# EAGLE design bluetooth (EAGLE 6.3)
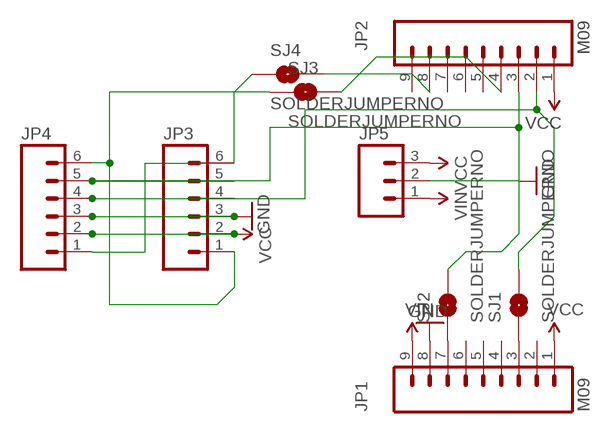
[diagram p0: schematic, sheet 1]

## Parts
JP1  M09  [1X09]
JP2  M09  [1X09]
JP3  M06LOCK  [1X06_LOCK]
JP4  M06LOCK  [1X06_LOCK]
JP5  M03PTH  [1X03]
SJ1  SOLDERJUMPERNO  [SJ_2S-NO]
SJ2  SOLDERJUMPERNO  [SJ_2S-NO]
SJ3  SOLDERJUMPERNO  [SJ_2S-NO]
SJ4  SOLDERJUMPERNO  [SJ_2S-NO]

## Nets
GND [POWER]: JP1.8 JP3.3 JP4.3 JP5.2
N$1: JP2.2 JP3.4 JP4.4 SJ1.2
N$2: JP2.3 JP3.5 JP4.5 SJ2.2
N$3: JP1.3 SJ1.1
N$4: JP1.7 SJ2.1
N$5: JP3.6 JP4.1 SJ4.1
N$6: JP3.1 JP4.6 SJ3.1
N$7: JP2.8 SJ4.2
N$8: JP2.4 SJ3.2
VCC: JP1.1 JP2.1 JP3.2 JP4.2 JP5.3
VIN: JP1.9 JP5.1
Unconnected: JP1.2 JP1.4 JP1.5 JP1.6 JP2.5 JP2.6 JP2.7 JP2.9

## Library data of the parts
JP1 JP2 = SparkFun:M09: Header 9 Standard 9-pin 0.1" header. Use with straight break away headers (SKU : PRT-00116), right angle break away headers (PRT-00553), swiss pins (PRT-00743), machine pins (PRT-00117), and female headers (PRT-00115).
JP3 JP4 = SparkFun-Connectors:M06: Header 6 Standard 6-pin 0.1" header. Use with straight break away headers (SKU : PRT-00116), right angle break away headers (PRT-00553), swiss pins (PRT-00743), machine pins (PRT-00117), and female headers (PRT-00115). Molex polarized connector foot print use with SKU : PRT-08094 with associated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
JP5 = SparkFun:M03: Header 3 Standard 3-pin 0.1" header. Use with straight break away headers (SKU : PRT-00116), right angle break away headers (PRT-00553), swiss pins (PRT-00743), machine pins (PRT-00117), and female headers (PRT-00115). Molex polarized connector foot print use with SKU : PRT-08232 with associated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
SJ1-SJ4 = SparkFun-Passives:SOLDERJUMPER: Solder Jumper

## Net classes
1 POWER: width 0.203 mm

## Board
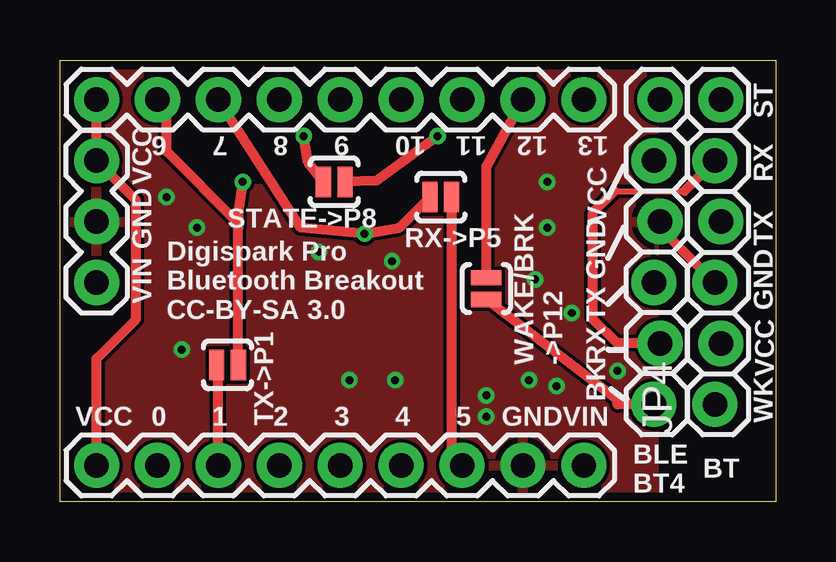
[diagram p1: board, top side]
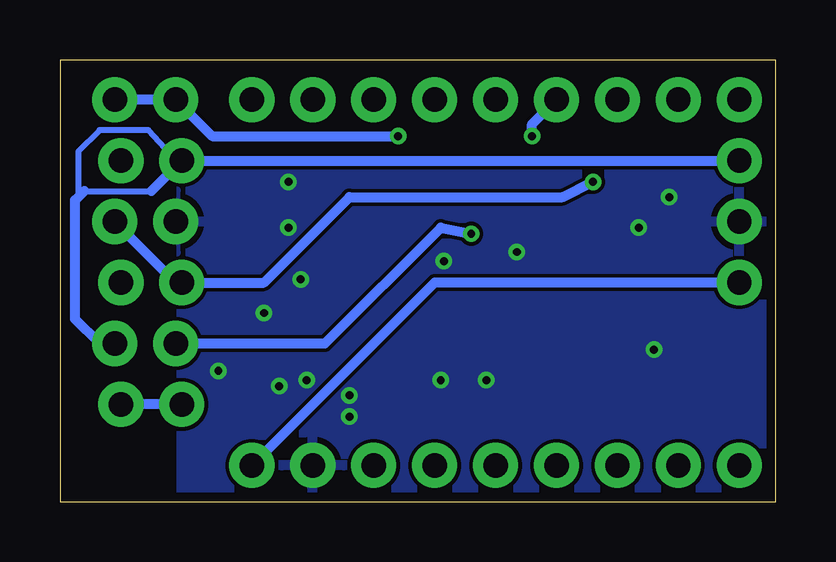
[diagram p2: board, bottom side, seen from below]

Size 29.84 x 18.41 mm. Coordinates in mm from the lower left corner, seen from the top.
Outline: 0,0 0,18.41 29.84,18.41 29.84,0 0,0
Copper layers (1*16): Top 0.0356mm / dielectric 1.5011mm / Bottom 0.0356mm
Design rules "eriks": minimum track width 6mil, minimum drill 13mil, track to track 6mil, track to pad 6mil, pad to pad 6mil, via to via 6mil, smd to smd 6mil, copper to edge 15mil, drill to drill 6mil, minimum pad ring 7mil, minimum via ring 7mil, stop-mask expansion 4mil, vias tented up to drill 20mil, thermal gap 10mil

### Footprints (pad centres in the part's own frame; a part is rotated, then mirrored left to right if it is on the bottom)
1X09 = drill 1.016 pad 1.88: 1 0,0; 2 2.54,0; 3 5.08,0; 4 7.62,0; 5 10.16,0; 6 12.7,0; 7 15.24,0; 8 17.78,0; 9 20.32,0
1X06_LOCK = drill 1.016 pad 1.88: 1 0,0; 2 2.54,-0.254; 3 5.08,0; 4 7.62,-0.254; 5 10.16,0; 6 12.7,-0.254
1X03 = drill 1.016 pad 1.88: 1 0,0; 2 2.54,0; 3 5.08,0
SJ_2S-NO = smd 0.635 x 1.27: 1 -0.45,0; 2 0.45,0

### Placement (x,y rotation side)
JP1  1.52,1.52 0 top
JP2  1.52,16.76 0 top
JP3  25.02,16.76 270 top
JP4  27.3,4.06 90 top
JP5  1.52,9.14 90 top
SJ1  6.99,5.71 0 top
SJ2  15.88,12.7 180 top
SJ3  11.43,13.34 180 top
SJ4  17.78,8.89 90 top

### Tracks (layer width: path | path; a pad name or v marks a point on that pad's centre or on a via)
GND  (via drill 0.33)
  Top 0.406: JP3.3 25.02,11.43 JP4.3
  other vias: 20.32,11.43 13.97,5.08 12.06,5.08 10.79,10.41 4.45,12.7 20.32,13.34 5.71,11.43 5.08,6.35 21.34,7.87 19.81,9.27 23.24,5.46 20.7,4.83 19.56,5.08 17.78,4.45 17.78,3.56 13.84,10.03
  pour Top: -2.54,24.13 -2.54,-1.91 24.77,-1.91 24.77,24.13
  pour Bottom: -2.54,23.5 -2.54,-2.54 24.77,-2.54 24.77,23.5
N$1  (via drill 0.33)
  Top 0.406: SJ1.2 7.43,11.43 | 7.43,11.43 7.43,11.62 4.45,14.61 4.45,16.38 JP2.2 | v7.62,13.34 7.43,12.06 7.43,11.43
  Bottom 0.406: JP4.4 25.02,9.14 JP3.4 21.34,9.14 17.78,12.7 8.89,12.7 v7.62,13.34
N$2  (via drill 0.33)
  Top 0.254: 23.11,12.95 26.04,12.95
  Top 0.406: JP2.3 10.03,11.43 v12.7,11.18 14.15,11.43 SJ2.2 | JP3.5 23.24,6.6 22.23,7.62 22.23,12.06 22.86,12.7 23.11,12.95 | 26.04,12.95 JP4.5
  Bottom 0.406: JP3.5 18.8,6.6 13.97,11.43 v12.7,11.18
N$3
  Top 0.406: JP1.3 6.6,5.65 SJ1.1
N$4
  Top 0.406: SJ2.1 16.32,1.96 JP1.7
N$5
  Top 0.406: JP3.6 23.24,4.06 23.24,4.25 SJ4.1
  Bottom 0.406: JP3.6 JP4.1
N$6  (via drill 0.33)
  Top 0.406: v15.75,15.24 13.21,13.39 SJ3.1
  Bottom 0.406: JP4.6 JP3.1 23.5,15.24 v15.75,15.24
N$7
  Top 0.406: SJ4.2 17.78,13.97 JP2.8
N$8  (via drill 0.33)
  Top 0.406: SJ3.2 10.35,14.15 v10.16,15.24
  Bottom 0.406: v10.16,15.24 10.16,15.75 JP2.4
VCC
  Top 0.406: JP1.1 1.52,5.97 3.17,7.62 3.17,12.57 JP5.3 JP2.1
  Bottom 0.254: 28.83,12.95 26.04,12.95 | 24.77,13.97 26.16,15.49 28.19,15.49 29.08,14.61 29.08,12.7
  Bottom 0.406: JP5.3 JP3.2 26.04,12.95 | JP4.2 28.19,6.6 29.21,7.62 29.21,12.57 29.08,12.7 28.83,12.95
VIN
  Bottom 0.406: JP5.1 14.22,9.14 JP1.9

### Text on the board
tPlace: ST | 6 | 7 | 8 | 9 | 10 | 11 | 12 | 13 | VCC | VCC | RX | GND | STATE->P8 | RX->P5 | TX | GND | VIN | Digispark Pro / Bluetooth Breakout / CC-BY-SA 3.0 | VCC | GND | TX | WAKE/BRK / ->P12 | RX | BK | VCC | 0 | 1 | 2 | TX->P1 | 3 | 4 | 5 | GND | VIN | WK | BT | BLE / BT4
